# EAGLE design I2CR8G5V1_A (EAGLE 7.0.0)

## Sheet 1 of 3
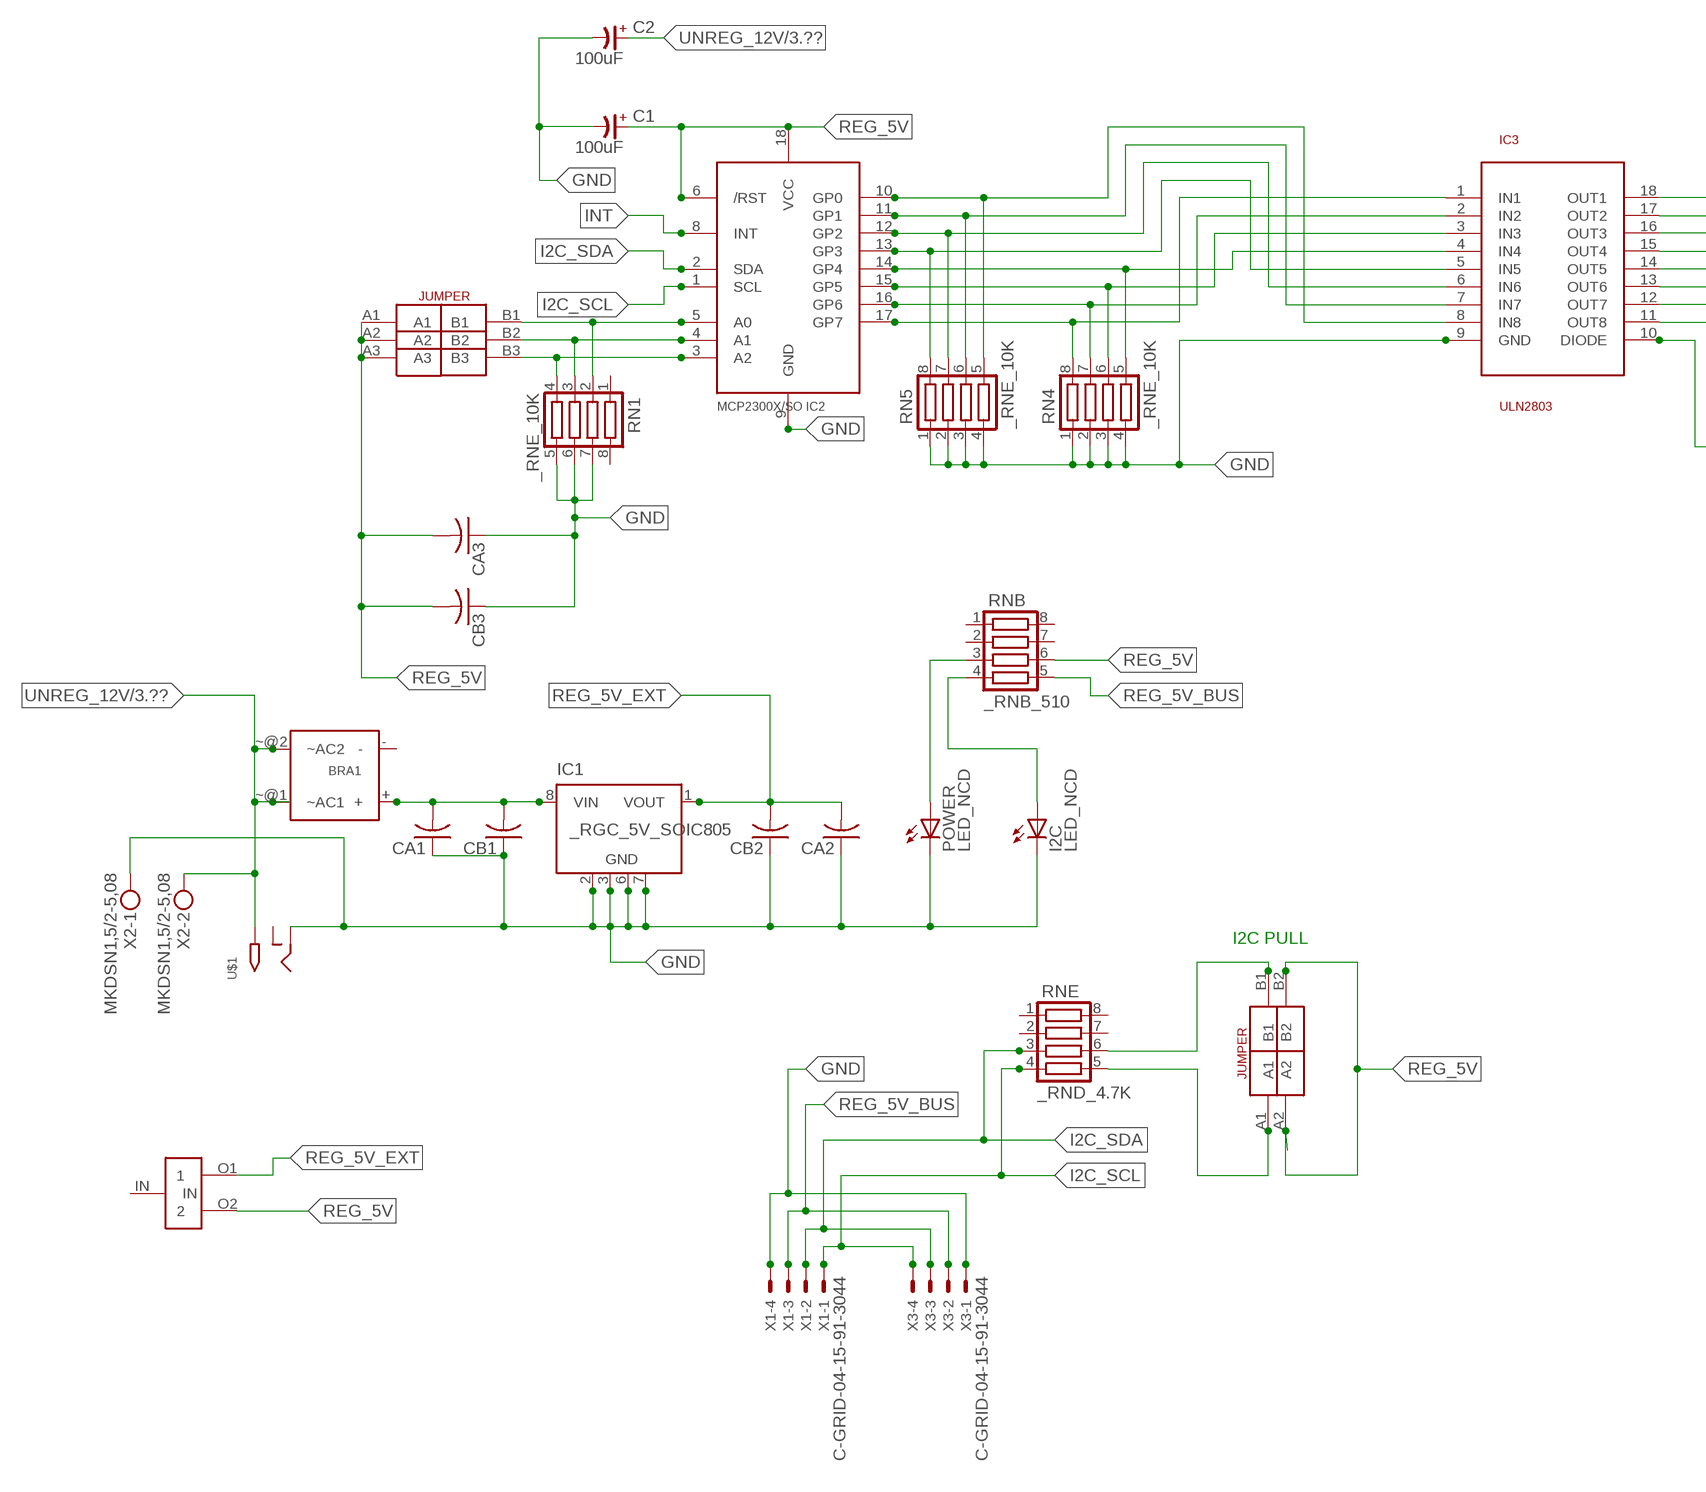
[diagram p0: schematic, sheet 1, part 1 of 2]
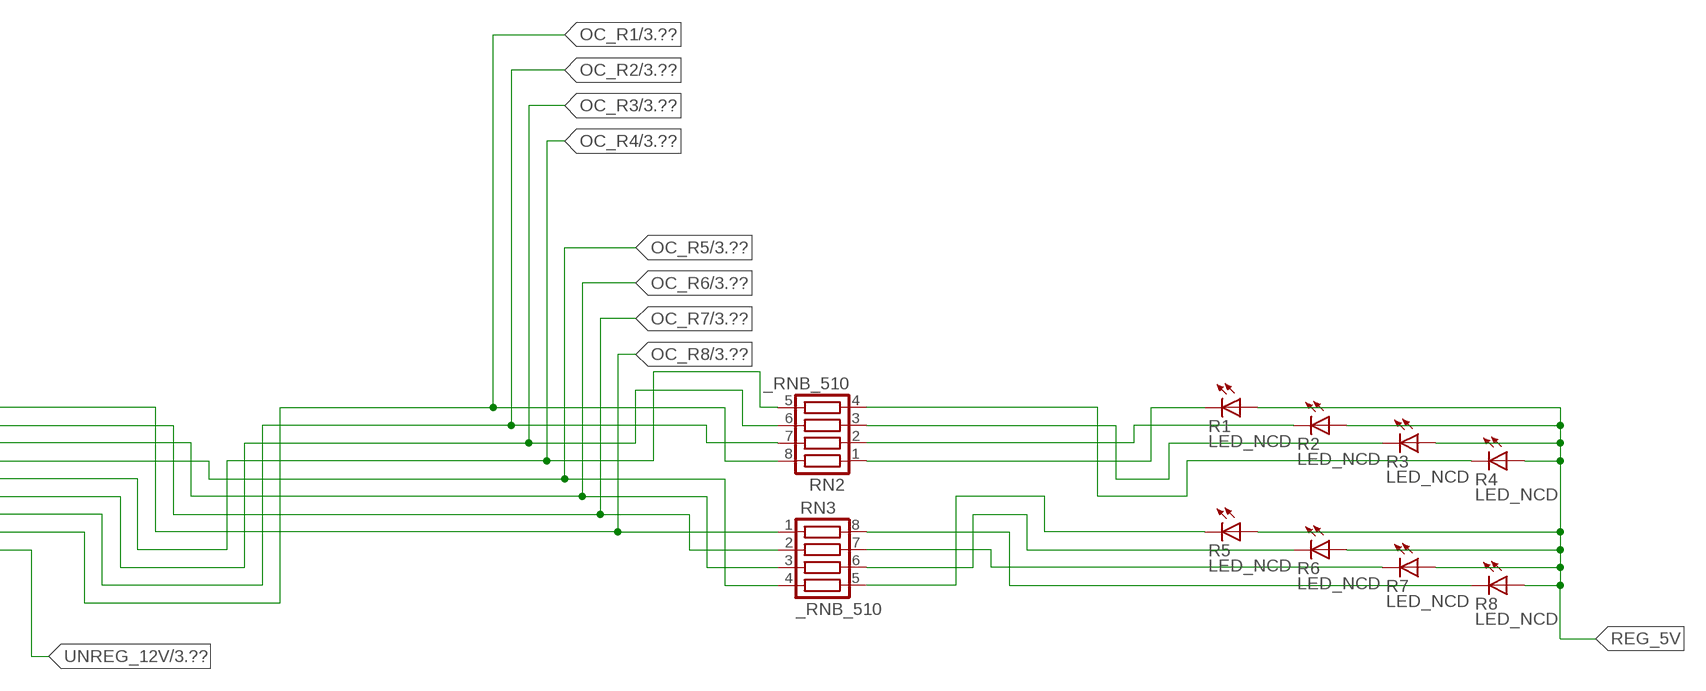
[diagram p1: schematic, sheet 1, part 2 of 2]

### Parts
BRA1  MB2S_  [MB2S]
C1  100uF  CP-E-025X060  [E-025X060]
C2  100uF  CP-E-025X060  [E-025X060]
CA1  CC1206KRX7R9BB104C1206K  [CC1206KRX7R9BB104]
CA2  CC1206KRX7R9BB104C1206K  [CC1206KRX7R9BB104]
CA3  CC1206KRX7R9BB104C1206K  [CC1206KRX7R9BB104]
CB1  TMK316F106ZL-TC1206K  [TMK316F106ZL-T]
CB2  TMK316F106ZL-TC1206K  [TMK316F106ZL-T]
CB3  TMK316F106ZL-TC1206K  [TMK316F106ZL-T]
I2C  LED_NCD  [CHIPLED_0603]
IC1  _RGC_5V_SOIC805  [_RGC_5V_SOIC8]
IC2  MCP2300X/SO  [SO18W]
IC3  ULN2803  [SO18L]
POWER  LED_NCD  [CHIPLED_0603]
R1  LED_NCD  [CHIPLED_0603]
R2  LED_NCD  [CHIPLED_0603]
R3  LED_NCD  [CHIPLED_0603]
R4  LED_NCD  [CHIPLED_0603]
R5  LED_NCD  [CHIPLED_0603]
R6  LED_NCD  [CHIPLED_0603]
R7  LED_NCD  [CHIPLED_0603]
R8  LED_NCD  [CHIPLED_0603]
RN1  _RNE_10K  [RNE]
RN2  _RNB_510  [RNB]
RN3  _RNB_510  [RNB]
RN4  _RNE_10K  [RNE]
RN5  _RNE_10K  [RNE]
RNB  _RNB_510  [RNB]
RNE  _RND_4.7K  [RND]
U$1  2.1MMJACK  [PJ-102A]
U$3  JUMPER_2X2  [JUMPER_2X2]
U$9  LINK_2  [LINK_2]
U$18  JUMPER_3X2  [JUMPER_3X2]
X1  C-GRID-04-15-91-3044  [15-91-04]
X2  MKDSN1,5/2-5,08  [MKDSN1,5/2-5,08]
X3  C-GRID-04-15-91-3044  [15-91-04]

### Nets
GND: C1.- C2.- CA1.1 CA2.1 CA3.1 CB1.1 CB2.1 CB3.1 I2C.C IC1.2(GND) IC1.3(GND) IC1.6(GND) IC1.7(GND) IC2.9(GND) IC3.9(GND) POWER.C RN1.5 RN1.6 RN1.7 RN4.1 RN4.2 RN4.3 RN4.4 RN5.1 RN5.2 RN5.3 RN5.4 U$1.RING X1.4 X2.1 X3.1
GP4: IC2.14(GP4) IC3.4(IN4) RN4.5
GP6: IC2.16(GP6) IC3.2(IN2) RN4.7
I2C_SCL: IC2.1(SCL) RNE.4 X1.1 X3.4
I2C_SDA: IC2.2(SDA) RNE.3 X1.2 X3.3
INT: IC2.8(INT)
N$1: BRA1.+ CA1.2 CB1.2 IC1.8(VIN)
N$2: POWER.A RNB.3
N$3: I2C.A RNB.4
N$4: RNE.5 U$3.A1
N$5: RNE.6 U$3.B1
N$6: IC2.5(A0) RN1.2 U$18.B1
N$7: IC2.4(A1) RN1.3 U$18.B2
N$8: IC2.3(A2) RN1.4 U$18.B3
N$20: R1.C RN2.1
N$21: IC2.12(GP2) IC3.6(IN6) RN5.7
N$22: IC2.11(GP1) IC3.7(IN7) RN5.6
N$23: IC2.10(GP0) IC3.8(IN8) RN5.5
N$29: R2.C RN2.2
N$30: R3.C RN2.3
N$31: R4.C RN2.4
N$32: R8.C RN3.8
N$81: R7.C RN3.7
N$82: R6.C RN3.6
N$83: R5.C RN3.5
N$89: IC2.13(GP3) IC3.5(IN5) RN5.8
N$93: IC2.15(GP5) IC3.3(IN3) RN4.6
N$94: IC2.17(GP7) IC3.1(IN1) RN4.8
OC_R1: IC3.11(OUT8) RN2.8 ; also sheet 3
OC_R2: IC3.12(OUT7) RN2.7 ; also sheet 3
OC_R3: IC3.13(OUT6) RN2.6 ; also sheet 3
OC_R4: IC3.14(OUT5) RN2.5 ; also sheet 3
OC_R5: IC3.15(OUT4) RN3.4 ; also sheet 3
OC_R6: IC3.16(OUT3) RN3.3 ; also sheet 3
OC_R7: IC3.17(OUT2) RN3.2 ; also sheet 3
OC_R8: IC3.18(OUT1) RN3.1 ; also sheet 3
REG_5V: C1.+ CA3.2 CB3.2 IC2.6(/RST) IC2.18(VCC) R1.A R2.A R3.A R4.A R5.A R6.A R7.A R8.A RNB.6 U$3.A2 U$3.B2 U$9.O2 U$18.A1 U$18.A2 U$18.A3
REG_5V_BUS: RNB.5 X1.3 X3.2
REG_5V_EXT: CA2.2 CB2.2 IC1.1(VOUT) U$9.O1
UNREG_12V: BRA1.~@1(~AC1) BRA1.~@2(~AC2) C2.+ IC3.10(DIODE) U$1.TIP X2.2 ; also sheet 3
Unconnected: BRA1.- IC1.4(NC) IC1.5(NC) RN1.1 RN1.8 RNB.1 RNB.2 RNB.7 RNB.8 RNE.1 RNE.2 RNE.7 RNE.8 U$1.RING_SW U$9.IN

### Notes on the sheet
- I2C PULL

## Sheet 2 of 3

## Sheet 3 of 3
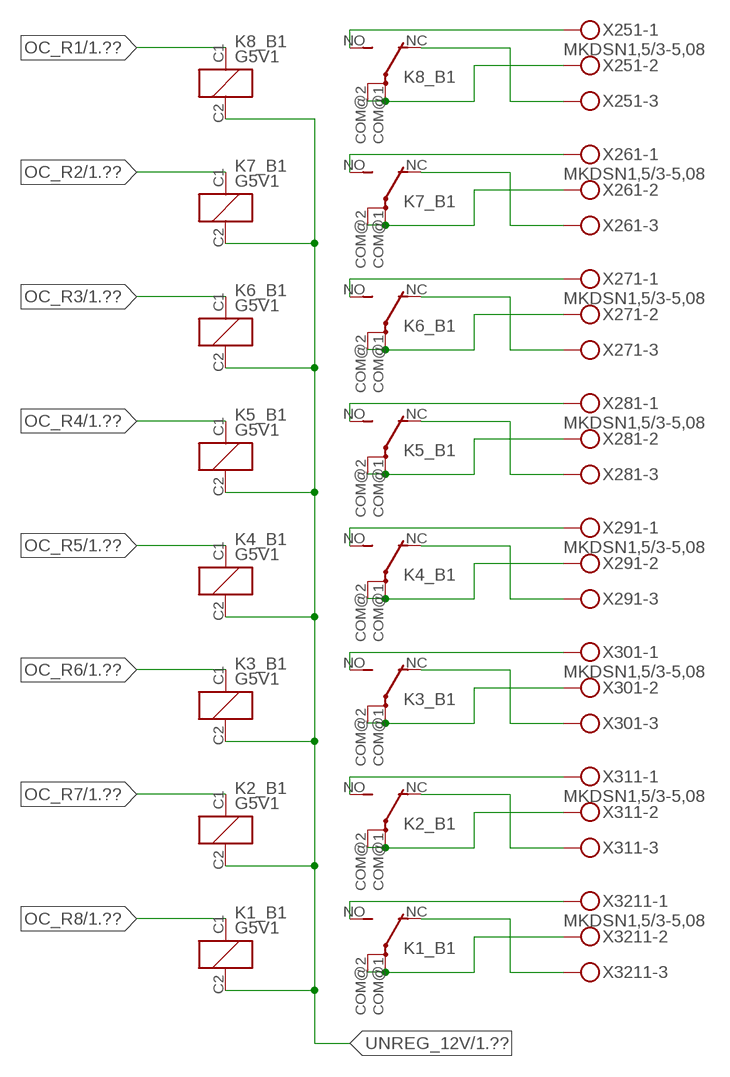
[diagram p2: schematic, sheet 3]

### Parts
K1_B1  G5V1  [G5V1]
K2_B1  G5V1  [G5V1]
K3_B1  G5V1  [G5V1]
K4_B1  G5V1  [G5V1]
K5_B1  G5V1  [G5V1]
K6_B1  G5V1  [G5V1]
K7_B1  G5V1  [G5V1]
K8_B1  G5V1  [G5V1]
X251  MKDSN1,5/3-5,08  [MKDSN1,5/3-5,08]
X261  MKDSN1,5/3-5,08  [MKDSN1,5/3-5,08]
X271  MKDSN1,5/3-5,08  [MKDSN1,5/3-5,08]
X281  MKDSN1,5/3-5,08  [MKDSN1,5/3-5,08]
X291  MKDSN1,5/3-5,08  [MKDSN1,5/3-5,08]
X301  MKDSN1,5/3-5,08  [MKDSN1,5/3-5,08]
X311  MKDSN1,5/3-5,08  [MKDSN1,5/3-5,08]
X3211  MKDSN1,5/3-5,08  [MKDSN1,5/3-5,08]

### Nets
N$203: K8_B1.COM@1(2:P) K8_B1.COM@2(2:P) X251.2
N$204: K8_B1.NC(2:O) X251.3
N$205: K8_B1.NO(2:S) X251.1
N$206: K7_B1.NO(2:S) X261.1
N$207: K6_B1.NO(2:S) X271.1
N$208: K7_B1.NC(2:O) X261.3
N$209: K7_B1.COM@1(2:P) K7_B1.COM@2(2:P) X261.2
N$210: K6_B1.NC(2:O) X271.3
N$211: K6_B1.COM@1(2:P) K6_B1.COM@2(2:P) X271.2
N$212: K5_B1.NC(2:O) X281.3
N$213: K5_B1.COM@1(2:P) K5_B1.COM@2(2:P) X281.2
N$214: K5_B1.NO(2:S) X281.1
N$215: K4_B1.NO(2:S) X291.1
N$216: K4_B1.NC(2:O) X291.3
N$217: K4_B1.COM@1(2:P) K4_B1.COM@2(2:P) X291.2
N$218: K3_B1.NO(2:S) X301.1
N$219: K3_B1.NC(2:O) X301.3
N$220: K3_B1.COM@1(2:P) K3_B1.COM@2(2:P) X301.2
N$221: K2_B1.NO(2:S) X311.1
N$222: K2_B1.NC(2:O) X311.3
N$223: K2_B1.COM@1(2:P) K2_B1.COM@2(2:P) X311.2
N$224: K1_B1.NO(2:S) X3211.1
N$225: K1_B1.NC(2:O) X3211.3
N$226: K1_B1.COM@1(2:P) K1_B1.COM@2(2:P) X3211.2
OC_R1: K8_B1.C1(1:C1) ; also sheet 1
OC_R2: K7_B1.C1(1:C1) ; also sheet 1
OC_R3: K6_B1.C1(1:C1) ; also sheet 1
OC_R4: K5_B1.C1(1:C1) ; also sheet 1
OC_R5: K4_B1.C1(1:C1) ; also sheet 1
OC_R6: K3_B1.C1(1:C1) ; also sheet 1
OC_R7: K2_B1.C1(1:C1) ; also sheet 1
OC_R8: K1_B1.C1(1:C1) ; also sheet 1
UNREG_12V: K1_B1.C2(1:C2) K2_B1.C2(1:C2) K3_B1.C2(1:C2) K4_B1.C2(1:C2) K5_B1.C2(1:C2) K6_B1.C2(1:C2) K7_B1.C2(1:C2) K8_B1.C2(1:C2) ; also sheet 1

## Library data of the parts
BRA1 = NCD_ULTIMATE_LIBRARY:MB2S: Bridge Rectifier BRA MB2S 200V 500ma Digikey MB2S-TPMSTR-ND/MB2S-TP
C1 C2 = NCD_ULTIMATE_LIBRARY:CP-: Capacitors All Kinds POLARIZED CAP
CA1-CA3 = NCD_ULTIMATE_LIBRARY:CC1206KRX7R9BB104: Capacitor CA .1uF 50V SMT C1206K CC1206KRX7R9BB104
CB1-CB3 = NCD_ULTIMATE_LIBRARY:TMK316F106ZL-T: Capacitor CB 10uF SMT 1206 TMK316F106ZL-T
I2C POWER = NCD_ULTIMATE_bhaskar:LED_NCD
IC1 = NCD_ULTIMATE_LIBRARY:_RGC_5V_SOIC8: Regulator Linear 5V Chip Positive VOLTAGE REGULATOR Digikey 497-7267-2-ND/L78L05CD13TR
IC2 = NCD_ULTIMATE_LIBRARY:MCP2300X: Semiconductor Port Expander I/O 8-Bit I2C MCP23008 Inexpensive i2c i/o expander - 8 general purpose i/o pins with optional pullups
IC3 = NCD_ULTIMATE_LIBRARY:ULN2803: Semiconductor 8 O.C. N-Channel Transistor Driver Digikey ULN2803AFWGCELTR-ND/ULN2803AFWG,C,EL
K1_B1 K2_B1 K3_B1 K4_B1 K5_B1 K6_B1 K7_B1 K8_B1 = NCD_ULTIMATE_LIBRARY:G5V1: RELAY 1 x switch, 0.5 A/125 V AC, 1 A/24 V DC , Omron
R1-R8 = NCD_ULTIMATE_LIBRARY:LED_NCD: LED Digikey 754-1132-2-ND/APT2012SRCPRV
RN1 RN4 RN5 = NCD_ULTIMATE_LIBRARY:_RNE_10K: Resistor Array RNE SMT 10K x 4 Single Resistor Source: http://www.ctscorp.com/components/Datasheets/CTSChipArrayDs.pdf Digikey 742C083103JPTR-ND/742C083103JP; OC_FARNELL: unknown; OC_NEWARK: unknown
RN2 RN3 RNB = NCD_ULTIMATE_LIBRARY:_RNB_510: Resistor Array RNB SMT 510 x 4 Single Resistor Source: http://www.ctscorp.com/components/Datasheets/CTSChipArrayDs.pdf Digikey 742C083511JPTR-ND/ 742C083511JP; OC_FARNELL: unknown; OC_NEWARK: unknown
RNE = NCD_ULTIMATE_LIBRARY:_RND_4.7K: Resistor Array RND SMT 4.7K x 4 Single Resistor Source: http://www.ctscorp.com/components/Datasheets/CTSChipArrayDs.pdf Digikey 742C083472JPTR-ND/742C083472JP; OC_FARNELL: unknown; OC_NEWARK: unknown
U$1 = NCD_ULTIMATE_CONNECTORS:2.1MMJACK: 2.1mm x 5.5mm DC jack with internal switch. Digikey part #PJ-102A, 4UCON part #05537 By microbuilder.eu
U$3 = NCD_ULTIMATE_CONNECTORS:JUMPER_2X2
U$9 = NCD_ULTIMATE_LIBRARY:LINK_2: PAD_top
U$18 = NCD_ULTIMATE_CONNECTORS:JUMPER_3X2
X1 X3 = NCD_ULTIMATE_CONNECTORS:C-GRID-04: CONNECTOR 4-Pos I2C wire to board 2.54 mm (0.100") pitch header Digikey WM1342-ND/0015912045; OC_FARNELL: unknown; OC_NEWARK: unknown
X2 = NCD_ULTIMATE_CONNECTORS:MKDSN1,5/2-5,08: MKDSN 1,5/ 2-5,08 Printklemme
X251 X261 X271 X281 X291 X301 X311 X3211 = NCD_ULTIMATE_CONNECTORS:MKDSN1,5/3-5,08: MKDSN 1,5/ 3-5,08 Printklemme Nennstrom: 13,5 A Nennspannung: 250 V Rastermaß: 5,08 mm Polzahl: 3 Anschlussart: Schraubanschluss Montage: Löten Anschlussrichtung Leiter/Platine: 0 ° Artikelnummer: 1729131 Source: http://eshop.phoenixcontact.com .. 1729131.pdf

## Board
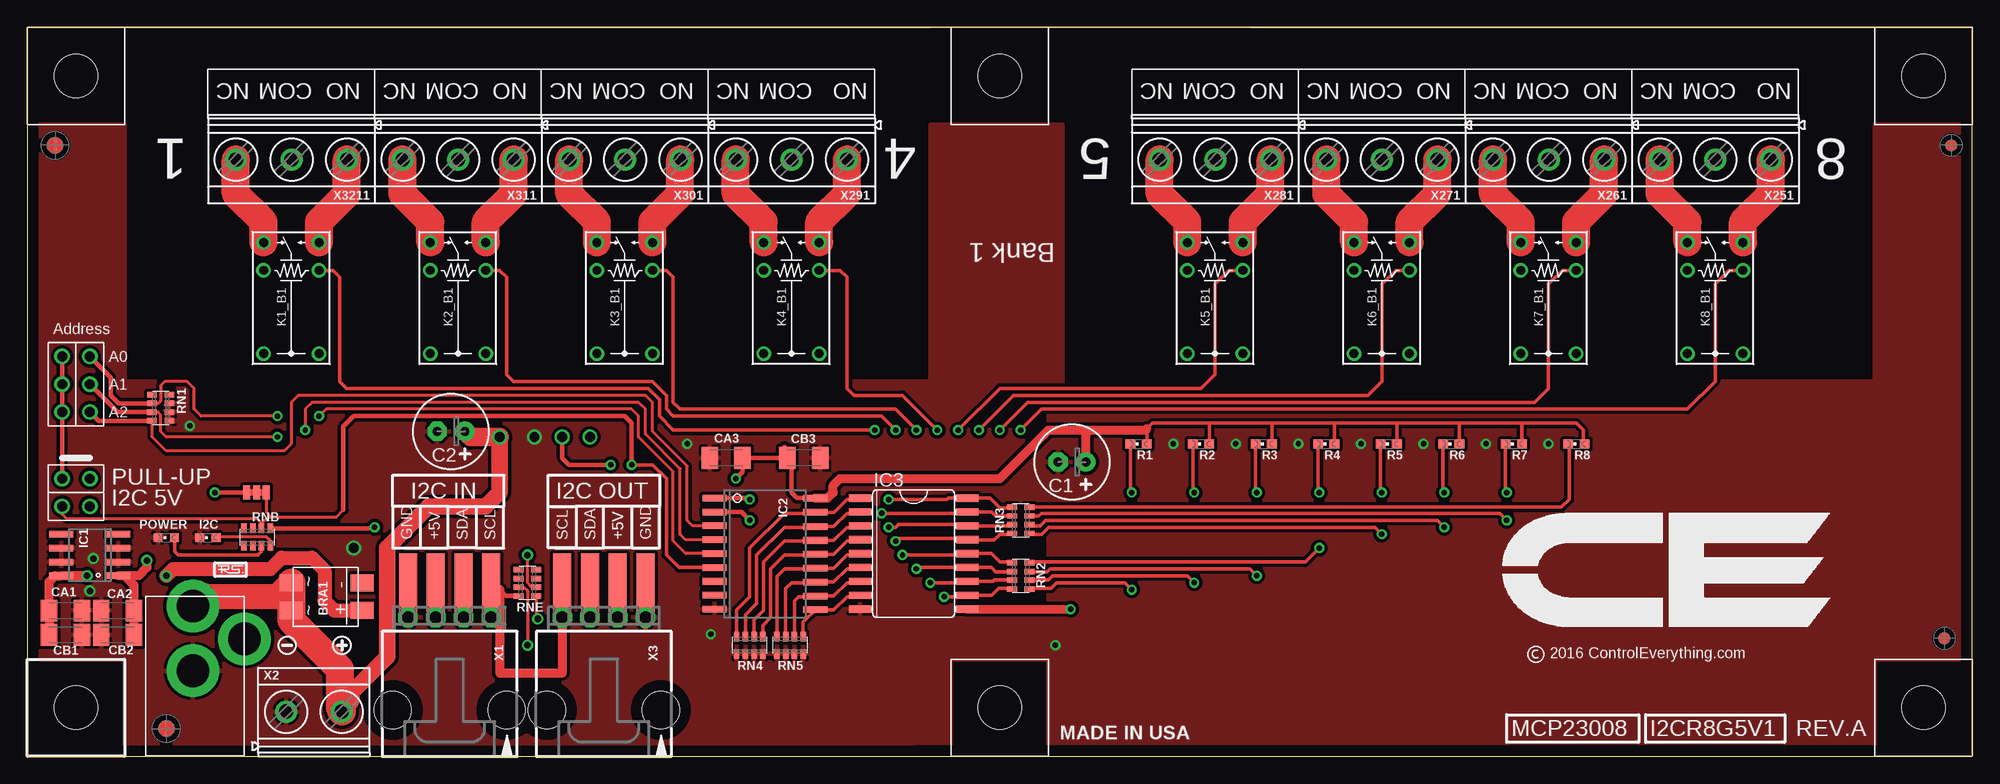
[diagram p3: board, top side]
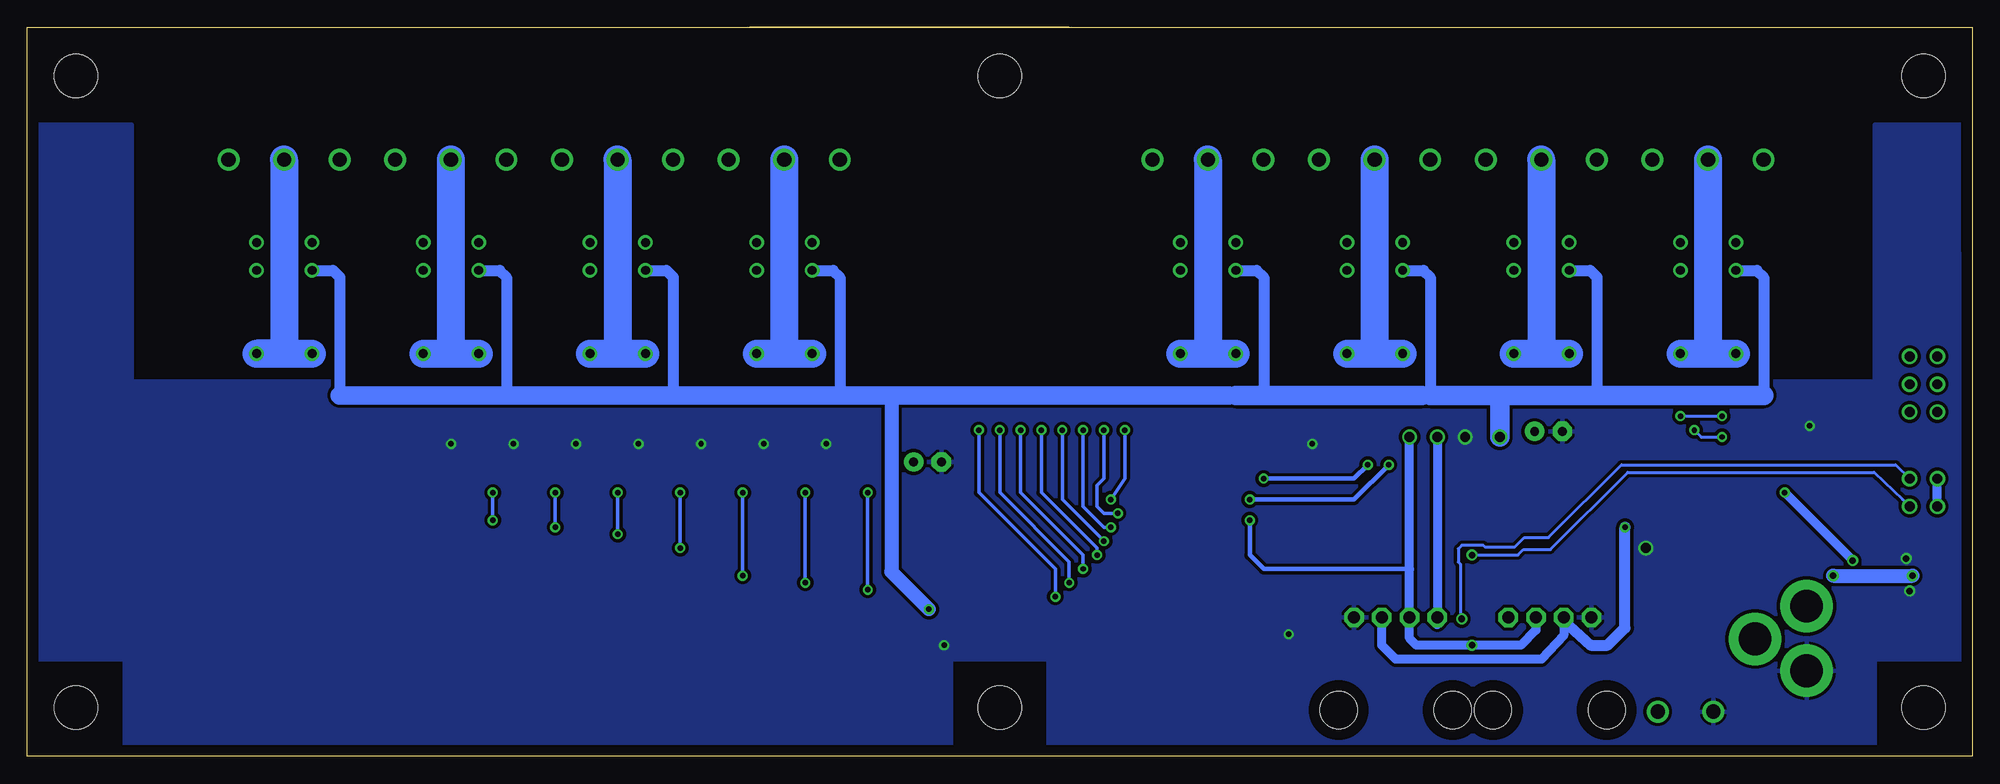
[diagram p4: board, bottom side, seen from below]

Size 177.8 x 66.67 mm. Coordinates in mm from the lower left corner, seen from the top.
Outline: 81.28,0 0,0 0,46.35
Outline: 81.28,0 82.53,0
Outline: 0,47.3 0,46.35
Outline: 81.28,0 177.8,0 177.8,66.67 0,66.67 0,46.35
Outline: 82.55,66.67 111.76,66.67
Copper layers (1*16): Top 0.035mm / dielectric 1.5mm / Bottom 0.035mm
Design rules "default": minimum track width 10mil, minimum drill 24mil, track to track 8mil, track to pad 8mil, pad to pad 8mil, via to via 8mil, smd to smd 8mil, copper to edge 40mil, drill to drill 8mil, minimum pad ring 10mil, minimum via ring 8mil, stop-mask expansion 4mil, vias tented up to drill 0mil, thermal gap 10mil
Holes 3.96 mm at 4.45,4.45

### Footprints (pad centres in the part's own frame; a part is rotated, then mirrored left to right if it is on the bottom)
MB2S = smd 1.55 x 2.1: + 0,-6.5; - 2.54,-6.5; ~@1 0,0; ~@2 2.54,0
E-025X060 = drill 0.813 pad 1.778: + -1.27,0 | drill 0.813 pad 1.778 octagon: - 1.27,0
CC1206KRX7R9BB104 = smd 1.5 x 2: 1 -1.5,0; 2 1.5,0
TMK316F106ZL-T = smd 1.5 x 2: 1 -1.5,0; 2 1.5,0
CHIPLED_0603 = smd 0.8 x 0.8: A 0,-0.75; C 0,0.75
_RGC_5V_SOIC8 = smd 0.6 x 2.2: 1 -1.905,-2.6; 2 -0.635,-2.6; 3 0.635,-2.6; 4 1.905,-2.6; 5 1.905,2.6; 6 0.635,2.6; 7 -0.635,2.6; 8 -1.905,2.6
SO18W = smd 0.6 x 2.2: 1 -4.445,-4.6; 2 -3.175,-4.6; 3 -1.905,-4.6; 4 -0.635,-4.6; 5 0.635,-4.6; 6 1.905,-4.6; 7 3.175,-4.6; 8 4.445,-4.6; 9 5.715,-4.6; 10 5.775,4.6; 11 4.505,4.6; 12 3.235,4.6; 13 1.965,4.6; 14 0.695,4.6; 15 -0.575,4.6; 16 -1.845,4.6; 17 -3.145,4.6; 18 -4.445,4.6
SO18L = smd 0.66 x 2.032: 1 -5.08,-4.902; 2 -3.81,-4.902; 3 -2.54,-4.902; 4 -1.27,-4.902; 5 0,-4.902; 6 1.27,-4.902; 7 2.54,-4.902; 8 3.81,-4.902; 9 5.08,-4.902; 10 5.08,4.902; 11 3.81,4.902; 12 2.54,4.902; 13 1.27,4.902; 14 0,4.902; 15 -1.27,4.902; 16 -2.54,4.902; 17 -3.81,4.902; 18 -5.08,4.902
G5V1 = drill 0.813: C1 -2.54,2.54; C2 -2.54,-2.54; COM@1 5.08,-2.54; COM@2 5.08,2.54; NC -5.08,-2.54; NO -5.08,2.54
CHIPLED_0603' = smd 0.8 x 0.876: A 0,-0.75; C 0,0.75
RNE = smd 0.5 x 0.9: 1 -1.2,-0.8; 2 -0.4,-0.8; 3 0.4,-0.8; 4 1.2,-0.8; 5 1.2,0.8; 6 0.4,0.8; 7 -0.4,0.8; 8 -1.2,0.8
RNB = smd 0.5 x 0.9: 1 -1.2,-0.8; 2 -0.4,-0.8; 3 0.4,-0.8; 4 1.2,-0.8; 5 1.2,0.8; 6 0.4,0.8; 7 -0.4,0.8; 8 -1.2,0.8
RND = smd 0.5 x 0.9: 1 -1.2,-0.8; 2 -0.4,-0.8; 3 0.4,-0.8; 4 1.2,-0.8; 5 1.2,0.8; 6 0.4,0.8; 7 -0.4,0.8; 8 -1.2,0.8
PJ-102A = drill 3 pad 4.8: RING 0.1,-3.39; RING_SW -4.6,-6.29; TIP 0.1,-9.29
JUMPER_2X2 = drill 0.9: A1 0,2.54; A2 0,0; B1 2.54,2.54; B2 2.54,0
PCB_MOUNTING_HOLE = hole 3.962: 4.445,4.445
LINK_2 = smd 1.27 x 0.635: IN 0,0; O1 0,0.889; O2 0,-0.889
JUMPER_3X2 = drill 0.9: A1 0,5.08; A2 0,2.54; A3 0,0; B1 2.54,5.08; B2 2.54,2.54; B3 2.54,0
15-91-04 = drill 1.1 pad 1.778 octagon: 1 -3.81,-7.62; 2 -1.27,-7.62; 3 1.27,-7.62; 4 3.81,-7.62 | smd 1.651 x 5.334: P1 -3.81,-10.795; P2 -1.27,-10.795; P3 1.27,-10.795; P4 3.81,-10.795 | hole 3.404: -5.207,0.838; 5.207,0.838
MKDSN1,5/2-5,08 = drill 1.3 pad 2: 1 -2.561,0.025; 2 2.519,0.025
MKDSN1,5/3-5,08 = drill 1.3 pad 2: 1 -7.641,0.025; 2 -2.561,0.025; 3 2.519,0.025

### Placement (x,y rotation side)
BRA1  24.13,13.34 90 top
C1  95.5,26.92 180 top
C2  38.73,29.72 180 top
CA1  3.49,13.34 180 top
CA2  8.26,13.34 0 top
CA3  63.88,27.3 0 top
CB1  3.49,11.11 180 top
CB2  8.26,11.11 0 top
CB3  70.99,27.3 180 top
I2C  16.51,20 90 top
IC1  5.71,18.41 90 top
IC2  67.44,19.18 270 top
IC3  81.03,18.54 270 top
K1_B1  24.13,41.91 270 top
K2_B1  39.37,41.91 270 top
K3_B1  54.61,41.91 270 top
K4_B1  69.85,41.91 270 top
K5_B1  108.58,41.91 270 top
K6_B1  123.83,41.91 270 top
K7_B1  139.06,41.91 270 top
K8_B1  154.31,41.91 270 top
POWER  12.7,20 90 top
R1  LED_NCD  [CHIPLED_0603']  101.6,28.57 90 top
R2  LED_NCD  [CHIPLED_0603']  107.31,28.57 90 top
R3  LED_NCD  [CHIPLED_0603']  113.03,28.57 90 top
R4  LED_NCD  [CHIPLED_0603']  118.75,28.57 90 top
R5  LED_NCD  [CHIPLED_0603']  124.46,28.57 90 top
R6  LED_NCD  [CHIPLED_0603']  130.18,28.57 90 top
R7  LED_NCD  [CHIPLED_0603']  135.89,28.57 90 top
R8  LED_NCD  [CHIPLED_0603']  141.6,28.57 90 top
RN1  12.19,31.88 270 top
RN2  90.81,16.51 90 top
RN3  90.81,21.59 270 top
RN4  66.04,10.16 0 top
RN5  69.72,10.16 0 top
RNB  21.02,20.07 0 top
RNE  45.72,15.88 270 top
U$1  15.24,4.45 180 top
U$3  3.17,25.4 270 top
U$4  [VISION_REF10]  175.26,10.79 270 top
U$5  PCB_MOUNTING_HOLE  [PCB_MOUNTING_HOLE]  177.8,57.78 90 top
U$6  PCB_MOUNTING_HOLE  [PCB_MOUNTING_HOLE]  93.34,0 90 top
U$7  PCB_MOUNTING_HOLE  [PCB_MOUNTING_HOLE]  93.34,57.78 90 top
U$8  PCB_MOUNTING_HOLE  [PCB_MOUNTING_HOLE]  8.89,57.78 90 top
U$9  20.95,24.13 90 top
U$10  [VISION_REF15]  12.7,2.54 0 top
U$11  PCB_MOUNTING_HOLE  [PCB_MOUNTING_HOLE]  177.8,0 90 top
U$12  PCB_MOUNTING_HOLE  [PCB_MOUNTING_HOLE]  177.8,57.78 90 top
U$15  [VISION_REF15]  2.54,55.88 270 top
U$18  3.17,31.5 0 top
U$21  [ICON_USA]  94.36,1.52 0 top
U$22  [ICON_MINUS]  23.75,10.16 180 top
U$24  [ICON_PLUS]  28.77,10.16 90 top
U$28  [VISION_REF10]  175.9,55.88 270 top
X1  38.61,5.08 180 top
X2  26.23,4.06 0 top
X3  52.7,5.08 180 top
X251  151.76,54.61 180 top
X261  136.53,54.61 180 top
X271  121.28,54.61 180 top
X281  106.05,54.61 180 top
X291  67.31,54.61 180 top
X301  52.07,54.61 180 top
X311  36.83,54.61 180 top
X3211  21.59,54.61 180 top

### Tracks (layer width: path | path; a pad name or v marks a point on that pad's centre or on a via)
GND  (via drill 0.5, 0.6, 0.9)
  Top 0.406: 34.8,12.38 X1.4
  Top 0.813: X3.1 56.52,12.06
  other vias: 5.71,15.11 6.03,18.1 46.35,29.21 29.84,19.05 14.86,30.23 62.48,11.18 127.64,28.57 93.98,10.16 133.35,28.57 139.06,28.57 121.92,28.57 116.2,28.57 110.49,28.57 104.78,28.57 60.33,28.57
  pour Bottom (isolate 0.305): 0.64,8.89 8.89,8.89 8.89,0 84.45,0 84.45,8.89 94.61,8.89 94.61,57.78 83.19,57.78 83.19,34.29 8.89,34.29 8.89,57.78 0.64,57.78
  pour Top (isolate 0.305): 0.64,8.89 8.89,8.89 8.89,0 84.45,0 84.45,8.89 94.61,8.89 94.61,57.78 82.55,57.78 82.55,34.29 8.89,34.29 8.89,57.78 0.64,57.78
  pour Top (isolate 0.305): 93.34,34.29 168.91,34.29 168.91,57.78 177.16,57.78 177.16,8.89 168.91,8.89 168.91,0 93.34,0
  pour Bottom (isolate 0.305): 93.34,0 93.34,34.29 168.28,34.29 168.28,57.78 177.16,57.78 177.16,8.89 168.91,8.89 168.91,0
GP4
  Top 0.305: RN4.5 67.24,11.99 67.94,12.7 67.94,17.14 69.22,18.41 71.97,18.41 IC2.14 73.73,18.48 74.93,19.68 76,19.68 IC3.4
GP6
  Top 0.305: RN4.7 65.64,12.94 66.67,13.97 66.67,18.41 69.22,20.95 71.97,20.95 IC2.16 73.73,21.02 74.93,22.23 76,22.23 IC3.2
I2C_SCL  (via drill 0.5, 0.9)
  Top 0.406: RNE.4 43.74,14.68 43.18,15.24 | IC2.1 65.91,23.62 v66.04,23.5 | v53.34,26.67 49.53,26.67 48.9,27.3 v48.9,29.21
  Top 0.813: X3.4 48.9,7.62 43.18,7.62 43.18,15.24 X1.1
  Bottom 0.406: v66.04,23.5 56.52,23.5 v53.34,26.67
  Bottom 0.813: v48.9,29.21 X3.4 48.9,12.06
I2C_SDA  (via drill 0.5, 0.6, 0.9)
  Top 0.254: RNE.3 45.36,15.47 45.72,15.11 v45.72,10.16
  Top 0.406: IC2.2 65.28,22.35 v66.04,21.59
  Top 0.61: X3.3 51.44,12.06 | X1.2 39.88,12.38
  Bottom 0.406: v66.04,21.59 66.04,18.41 64.77,17.14 51.44,17.14 | 39.88,12.38 X1.2
  Bottom 0.813: 39.88,12.38 39.88,11.56 41.27,10.16 v45.72,10.16 50.8,10.16 51.44,10.79 51.44,12.06 X3.3 51.44,17.14 v51.44,29.21
N$1  (via drill 0.6)
  Top 0.813: CB1.2 CA1.2 1.99,15.96 2.54,16.51 IC1.8 v5.46,16.51
  Top 1.27: v12.7,16.51 13.34,17.14 22.23,17.14 23.24,18.16 26.04,18.16 27.18,17.02 27.18,14.22 28.07,13.34 BRA1.+
  Bottom 1.27: v12.7,16.51 v5.46,16.51
N$2
  Top 0.305: RNB.3 21.4,18.95 21.4,18.7 21.12,18.41 13.78,18.41 13.45,18.74 POWER.A
N$3
  Top 0.254: 22.23,18.95 22.23,19.74 21.9,20.07 16.94,20.07
  Top 0.305: RNB.4 22.23,18.95 | 16.94,20.07 I2C.A
N$4  (via drill 0.6)
  Top 0.254: RNE.5 46.52,12.6 v46.67,12.57
  Bottom 0.254: U$3.A1 6.99,26.67 32.07,26.67 38.73,20 40.96,20 41.85,19.11 44.51,19.11 44.7,19.3 46.67,19.3 46.99,18.99 46.99,17.78 46.8,17.59 46.8,12.7 v46.67,12.57
N$5  (via drill 0.6)
  Top 0.254: RNE.6 46.12,15.47 45.72,15.88 v45.72,18.41
  Bottom 0.254: v45.72,18.41 41.53,18.41 41.02,18.92 38.54,18.92 31.5,25.97 8.95,25.97 6.35,23.5 U$3.B1
N$6  (via drill 0.5)
  Top 0.254: IC2.5 60.2,18.54 59.05,19.68 59.05,26.04 55.88,29.21 55.88,31.11 55.24,31.75 27.3,31.75 v26.67,31.11 | v22.86,31.11 15.88,31.11 15.24,31.75 15.24,33.66 14.61,34.29 12.57,34.29 12.19,33.91 12.19,32.51 11.94,32.26 11.41,32.26 RN1.2
  Top 0.406: RN1.2 8.36,32.28 7.62,33.02 7.62,34.67 U$18.B1
  Bottom 0.254: v26.67,31.11 v22.86,31.11
N$7  (via drill 0.5)
  Top 0.254: IC2.4 60.2,19.81 59.69,20.32 59.69,26.29 56.52,29.46 56.52,31.75 55.88,32.38 26.04,32.38 25.4,31.75 v25.4,29.84 | v22.86,29.21 12.7,29.21 12.19,29.72 12.19,31.24 11.94,31.5 11.41,31.5 RN1.3
  Top 0.406: RN1.3 8.27,31.48 U$18.B2
  Bottom 0.254: v25.4,29.84 24.77,29.21 v22.86,29.21
N$8
  Top 0.254: IC2.3 60.83,21.08 60.33,21.59 60.33,26.54 57.15,29.72 57.15,32.38 56.52,33.02 24.77,33.02 24.13,32.38 24.13,28.57 23.5,27.94 12.7,27.94 11.43,29.21 11.43,30.64 RN1.4
  Top 0.406: RN1.4 6.53,30.68 U$18.B3
N$20  (via drill 0.5)
  Top 0.305: R1.C 100.85,24.25 v100.97,24.13 | v100.97,15.24 100.33,15.88 94.11,15.88 93.6,15.37 91.66,15.37 RN2.1
  Bottom 0.305: v100.97,24.13 v100.97,15.24
N$21
  Top 0.305: RN5.7 69.32,15.35 69.85,15.88 71.97,15.88 IC2.12 73.73,15.94 74.93,17.14 76,17.14 IC3.6
N$22
  Top 0.305: RN5.6 70.12,14.24 70.48,14.61 71.97,14.61 IC2.11 73.73,14.67 74.93,15.88 76,15.88 IC3.7
N$23
  Top 0.254: 71.97,13.34 IC2.10
  Top 0.305: RN5.5 70.92,12.29 IC2.10 73.73,13.4 74.93,14.61 76,14.61 IC3.8
N$29  (via drill 0.5)
  Top 0.305: R2.C 106.56,24.25 v106.68,24.13 | v106.68,15.88 106.05,16.51 93.73,16.51 93.34,16.13 91.62,16.13 RN2.2
  Bottom 0.305: v106.68,24.13 v106.68,15.88
N$30  (via drill 0.5)
  Top 0.305: R3.C 112.28,24.25 v112.39,24.13 | v112.39,16.51 111.76,17.14 93.47,17.14 93.22,16.89 91.62,16.89 RN2.3
  Bottom 0.305: v112.39,24.13 v112.39,16.51
N$31  (via drill 0.5)
  Top 0.305: R4.C 118,24.25 v118.11,24.13 | v118.11,19.05 116.84,17.78 91.67,17.78 RN2.4
  Bottom 0.305: v118.11,24.13 v118.11,19.05
N$32
  Top 0.305: RN3.8 140.26,22.79 140.97,23.5 140.97,28.46 R8.C
N$81  (via drill 0.5)
  Top 0.305: R7.C 135.14,24.25 v135.25,24.13 | v135.25,21.59 134.62,22.23 92.71,22.23 92.46,21.97 91.62,21.97 RN3.7
  Bottom 0.305: v135.25,24.13 v135.25,21.59
N$82  (via drill 0.5)
  Top 0.305: R6.C 129.43,24.25 v129.54,24.13 | v129.54,20.95 128.91,21.59 93.09,21.59 92.58,21.08 91.71,21.08 RN3.6
  Bottom 0.305: v129.54,24.13 v129.54,20.95
N$83  (via drill 0.5)
  Top 0.305: R5.C 123.71,24.25 v123.83,24.13 | v123.83,20.32 123.19,20.95 93.34,20.95 92.71,20.32 91.67,20.32 RN3.5
  Bottom 0.305: v123.83,24.13 v123.83,20.32
N$89
  Top 0.305: RN5.8 68.52,16.45 69.22,17.14 71.97,17.14 IC2.13 73.73,17.21 74.93,18.41 76,18.41 IC3.5
N$93
  Top 0.305: RN4.6 66.44,12.46 67.31,13.34 67.31,17.78 69.22,19.68 71.97,19.68 IC2.15 73.73,19.75 74.93,20.95 76,20.95 IC3.3
N$94
  Top 0.305: RN4.8 64.84,13.4 66.04,14.61 66.04,19.05 69.22,22.23 71.94,22.23 IC2.17 73.76,22.32 74.93,23.5 76,23.5 IC3.1
N$203
  Bottom 2.54: X251.2 154.33,36.85 154.31,36.83 K8_B1.COM@2 K8_B1.COM@1
N$204
  Top 2.54: K8_B1.NC 151.76,48.9 149.22,51.44 149.22,54.56 X251.3
N$205
  Top 2.54: K8_B1.NO 156.84,48.9 159.38,51.44 159.38,54.56 X251.1
N$206
  Top 2.54: K7_B1.NO 141.6,48.9 144.15,51.44 144.15,54.56 X261.1
N$207
  Top 2.54: K6_B1.NO 126.36,48.9 128.91,51.44 128.91,54.56 X271.1
N$208
  Top 2.54: K7_B1.NC 136.53,48.9 133.99,51.44 133.99,54.56 X261.3
N$209
  Bottom 2.54: K7_B1.COM@2 139.06,36.83 | 139.06,36.83 K7_B1.COM@1 | X261.2 139.09,36.85 139.06,36.83
N$210
  Top 2.54: K6_B1.NC 121.28,48.9 118.75,51.44 118.75,54.56 X271.3
N$211
  Bottom 2.54: K6_B1.COM@2 123.83,36.83 | 123.83,36.83 K6_B1.COM@1 | X271.2 123.85,36.85 123.83,36.83
N$212
  Top 2.54: K5_B1.NC 106.05,48.9 103.5,51.44 103.5,54.56 X281.3
N$213
  Bottom 2.54: K5_B1.COM@2 108.58,36.83 | 108.58,36.83 K5_B1.COM@1 | X281.2 108.61,36.85 108.58,36.83
N$214
  Top 2.54: K5_B1.NO 111.12,48.9 113.67,51.44 113.67,54.56 X281.1
N$215
  Top 2.54: K4_B1.NO 72.39,48.9 74.93,51.44 74.93,54.56 X291.1
N$216
  Top 2.54: K4_B1.NC 67.31,48.9 64.77,51.44 64.77,54.56 X291.3
N$217
  Bottom 2.54: K4_B1.COM@2 69.85,36.83 | 69.85,36.83 K4_B1.COM@1 | X291.2 69.87,36.85 69.85,36.83
N$218
  Top 2.54: K3_B1.NO 57.15,48.9 59.69,51.44 59.69,54.56 X301.1
N$219
  Top 2.54: K3_B1.NC 52.07,48.9 49.53,51.44 49.53,54.56 X301.3
N$220
  Bottom 2.54: K3_B1.COM@2 54.61,36.83 | 54.61,36.83 K3_B1.COM@1 | X301.2 54.63,36.85 54.61,36.83
N$221
  Top 2.54: K2_B1.NO 41.91,48.9 44.45,51.44 44.45,54.56 X311.1
N$222
  Top 2.54: K2_B1.NC 36.83,48.9 34.29,51.44 34.29,54.56 X311.3
N$223
  Bottom 2.54: K2_B1.COM@2 39.37,36.83 | 39.37,36.83 K2_B1.COM@1 | X311.2 39.39,36.85 39.37,36.83
N$224
  Top 2.54: K1_B1.NO 26.67,48.9 29.21,51.44 29.21,54.56 X3211.1
N$225
  Top 2.54: K1_B1.NC 21.59,48.9 19.05,51.44 19.05,54.56 X3211.3
N$226
  Bottom 2.54: K1_B1.COM@2 24.13,36.83 | 24.13,36.83 K1_B1.COM@1 | X3211.2 24.15,36.85 24.13,36.83
OC_R1  (via drill 0.5)
  Top 0.305: RN2.8 89.95,15.37 88.77,15.37 88.14,14.73 IC3.11 85.8,14.61 v83.82,14.61 | v90.81,29.84 92.71,31.75 151.76,31.75 154.31,34.29 154.31,43.18 155.57,44.45 K8_B1.C1
  Bottom 0.305: v90.81,29.84 90.81,24.13 83.82,17.14 v83.82,14.61
OC_R2  (via drill 0.5)
  Top 0.305: RN2.7 89.99,16.13 88.39,16.13 88.27,16 IC3.12 85.8,15.88 v82.55,15.88 | v88.9,29.84 91.44,32.38 137.79,32.38 139.06,33.66 139.06,43.18 140.34,44.45 K7_B1.C1
  Bottom 0.305: v88.9,29.84 88.9,24.13 82.55,17.78 v82.55,15.88
OC_R3  (via drill 0.5)
  Top 0.305: RN2.6 89.99,16.89 88.52,16.89 88.14,17.27 IC3.13 81.53,17.27 81.41,17.14 v81.28,17.14 | v87,29.84 90.17,33.02 122.56,33.02 123.83,34.29 123.83,43.18 125.09,44.45 K6_B1.C1
  Bottom 0.305: v87,29.84 87,24.13 81.28,18.41 v81.28,17.14
OC_R4  (via drill 0.5)
  Top 0.305: RN2.5 89.94,17.78 88.9,17.78 88.14,18.54 IC3.14 85.8,18.41 v80.01,18.41 | v85.09,29.84 88.9,33.66 107.31,33.66 108.58,34.92 108.58,43.18 109.86,44.45 K5_B1.C1
  Bottom 0.305: v85.09,29.84 85.09,24.13 80.01,19.05 v80.01,18.41
OC_R5  (via drill 0.5)
  Top 0.305: RN3.4 89.94,20.32 88.9,20.32 88.39,19.81 IC3.15 85.8,19.94 79.63,19.94 v79.38,19.68 | v83.19,29.84 80.01,33.02 75.56,33.02 74.93,33.66 74.93,43.81 74.3,44.45 K4_B1.C1
  Bottom 0.305: v83.19,29.84 83.19,23.5 v79.38,19.68
OC_R6  (via drill 0.5)
  Top 0.305: RN3.3 89.9,21.08 IC3.16 85.8,21.21 79.63,21.21 79.38,20.95 v78.74,20.95 | v81.28,29.84 79.38,31.75 59.69,31.75 59.05,32.38 59.05,43.81 58.42,44.45 K3_B1.C1
  Bottom 0.305: v81.28,29.84 81.28,22.86 79.38,20.95 v78.74,20.95
OC_R7  (via drill 0.5)
  Top 0.305: RN3.2 89.99,21.97 88.52,21.97 88.14,22.35 IC3.17 85.8,22.23 v78.11,22.23 | v79.38,29.84 78.11,31.11 59.05,31.11 58.42,31.75 58.42,33.02 57.15,34.29 44.45,34.29 43.81,34.92 43.81,43.81 43.18,44.45 K2_B1.C1
  Bottom 0.305: v79.38,29.84 79.38,25.4 80.01,24.77 80.01,22.86 79.38,22.23 v78.11,22.23
OC_R8  (via drill 0.5)
  Top 0.305: RN3.1 89.95,22.73 88.9,22.73 88.01,23.62 IC3.18 84.2,23.62 84.07,23.5 v78.74,23.5 | v77.47,29.84 59.05,29.84 57.78,31.11 57.78,32.64 56.77,33.66 29.21,33.66 28.57,34.29 28.57,43.81 27.94,44.45 K1_B1.C1
  Bottom 0.305: v77.47,29.84 77.47,25.4 v78.74,23.5
REG_5V  (via drill 0.5)
  Top 0.254: RNB.6 21.42,21.29 | 21.42,21.29 22.04,21.91 22.23,21.91 | 21.42,21.29 20.99,21.72 3.62,21.72 3.17,22.16 U$3.B2 | 22.23,21.91 28.26,21.91 28.89,22.54 | U$9.O2 21.84,22.29 22.23,21.91
  Top 0.305: v55.24,26.67 57.15,26.67 58.42,25.4 58.42,18.41 59.56,17.27 IC2.6 | R1.A 102.35,29.96 102.87,30.48 107.95,30.48 | 107.95,30.48 113.67,30.48 | 113.67,30.48 119.38,30.48 | 119.38,30.48 125.09,30.48 | 125.09,30.48 130.81,30.48 | 130.81,30.48 136.53,30.48 | 136.53,30.48 141.6,30.48 142.24,29.84 142.24,28.69 R8.A | R7.A 136.64,30.36 136.53,30.48 | R6.A 130.93,30.36 130.81,30.48 | R5.A 125.21,30.36 125.09,30.48 | R4.A 119.5,30.36 119.38,30.48 | R3.A 113.78,30.36 113.67,30.48 | R2.A 108.06,30.36 107.95,30.48
  Top 0.406: U$18.A1 U$18.A2 U$18.A3 U$3.A2 | IC2.18 70.36,23.62 69.85,24.13 69.85,27.58 CB3.2 CA3.2 65.38,26.01 v64.77,25.4 | 62.71,17.14 IC2.6 | 28.89,22.54 28.89,30.16 29.84,31.11 54.61,31.11 55.24,30.48 v55.24,26.67
  Top 0.61: 69.22,28.22 CB3.2
  Top 0.813: IC2.18 73.15,23.62 73.66,24.13 73.66,24.77 74.3,25.4 88.9,25.4 93.34,29.84 97.16,29.84 | 97.16,29.84 102.23,29.84 102.35,29.96 | C1.+ 96.77,29.46 97.16,29.84
  Bottom 0.406: v64.77,25.4 56.52,25.4 v55.24,26.67
  Bottom 0.813: U$3.B2 U$3.A2
REG_5V_BUS  (via drill 0.5)
  Top 0.406: RNB.5 31.2,20.87 v31.75,20.95
  Top 0.61: X1.3 37.34,12.38 | X3.2 53.98,12.06
  Bottom 0.406: 37.34,12.38 X1.3 | 53.98,12.06 X3.2
  Bottom 0.813: 37.34,12.38 37.34,11.05 39.37,8.89 52.7,8.89 53.98,10.16 53.98,12.06
  Bottom 1.016: 37.34,12.38 34.86,10.16 33.34,10.16 31.75,11.75 v31.75,20.95
REG_5V_EXT  (via drill 0.5, 0.6)
  Top 0.406: U$9.O1 v17.14,24.13
  Top 0.813: CB2.2 CA2.2 9.76,15.64 8.89,16.51 | 8.89,16.51 IC1.1 | v10.92,17.91 10.92,17.27 10.16,16.51 8.89,16.51
  Bottom 0.813: v17.14,24.13 v10.92,17.91
UNREG_12V  (via drill 0.5, 0.9)
  Top 0.762: v95.38,13.46 IC3.10
  Top 1.524: v43.18,29.21 43.18,24.13 41.91,22.86 36.7,22.86 32.89,19.05 32.89,9.08 29.11,5.3 28.57,4.76
  Top 1.676: v43.18,29.21 40.51,29.21 C2.+
  Top 2.286: BRA1.~@2 22.86,14.61 16.01,14.61
  Top 2.54: 16.01,14.61 U$1.TIP | X2.2 28.55,4.45 28.57,4.76 | BRA1.~@2 BRA1.~@1 24.13,12.45 28.57,8 28.57,5.84 29.11,5.3
  Bottom 1.016: K1_B1.C2 19.68,44.45 19.05,43.81 19.05,33.02 | K2_B1.C2 34.92,44.45 34.29,43.81 34.29,33.02 | K3_B1.C2 50.16,44.45 49.53,43.81 49.53,33.02 50.29,33.02 | K4_B1.C2 65.41,44.45 64.77,43.81 64.77,33.02 | 67.31,33.02 67.94,33.02 | K5_B1.C2 104.14,44.45 103.5,43.81 103.5,33.66 104.14,33.02 | 98.81,33.02 99.06,33.02 | K6_B1.C2 119.38,44.45 118.75,43.81 118.75,33.66 118.11,33.02 | 116.84,33.02 116.59,33.02 | K7_B1.C2 134.62,44.45 133.99,43.81 133.99,33.02 | 134.37,33.02 134.62,33.02 | K8_B1.C2 149.86,44.45 149.22,43.81 149.22,33.02
  Bottom 1.27: 98.81,33.02 98.81,16.89 v95.38,13.46
  Bottom 1.676: 67.94,33.02 98.81,33.02 | 99.06,33.02 104.14,33.02 116.59,33.02 | 116.84,33.02 118.11,33.02 133.99,33.02 134.37,33.02 | 134.62,33.02 149.22,33.02
  Bottom 1.778: v43.18,29.21 43.18,33.02 | 43.18,33.02 34.29,33.02 19.05,33.02 | 49.53,33.02 43.18,33.02 | 67.31,33.02 64.77,33.02 50.29,33.02

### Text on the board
tNames: NC | COM | NO | NC | COM | NO | NC | COM | NO | NC | COM | NO | NC | COM | NO | NC | COM | NO | NC | COM | NO | NC | COM | NO | 1 | 4 | 5 | 8 | Bank 1 | Address | A0 | A1 | A2 | PULL-UP | I2C IN | I2C OUT | I2C 5V | GND | +5V | SDA | SCL | SCL | SDA | +5V | +5V | GND | 2016 ControlEverything.com | MCP23008 | I2CR8G5V1 | REV.A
